TYPE "ST_AcyclicReadRequest"
VERSION : 0.1


  STRUCT
   byServiceID : BYTE ;	//Service ID |  0x10 = Read object acyclic
   dwMessageID : DWORD ;	//Message ID | Free usable message ID of the application | Can be set from the cl
   dwDataLength : DWORD ;	//Data length | Must be 0x04 in this request (Object index, Sub index, Reserved)
   byAcknowledge : BYTE ;	//Acknowledge | Can be set to 0x00 in this request
   dwReadType : DWORD ;	//Read type | 0x00 = Single read object | Read object with one sub index (e.g. 0x
   wIndex : WORD ;	//Index | Index of the object to be read
   bySubIndex : BYTE ;	//Sub index | Sub index of the object to be read
   byReserved : BYTE ;	//Reserved | Can be set to 0x00 in this request
  END_STRUCT ;
END_TYPE

